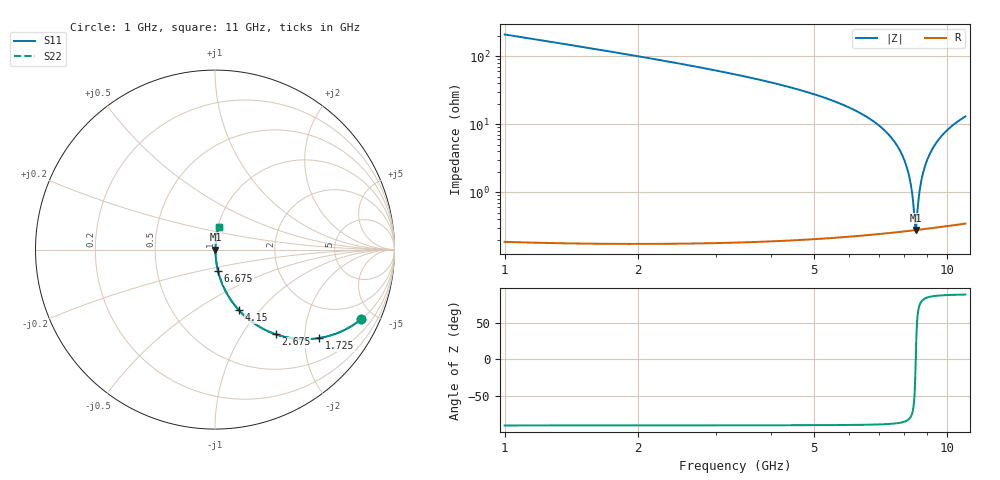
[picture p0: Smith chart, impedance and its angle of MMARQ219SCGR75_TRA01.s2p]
! MMARQ219SCGR75_TRA01  S-PARAMETER MODEL  ( General Type )
! Model Generated by TAIYO YUDEN Corporation (http://www.ty-top.com)
! Version 1.0
! TAIYO YUDEN Control No. 180601
! Copyright(c) 2018 TAIYO YUDEN CO.,LTD. All Rights Reserved.
! Product Description (link to TY-COMPAS)
! https://ds.yuden.co.jp/TYCOMPAS/or/detail?pn=MMARQ219SCGR75BTRA01&u=M
! Products Name : Multilayer Ceramic Capacitors
! Characteristics :
!  Capacitance : 0.75 pF , Rated Voltage : 250V , TCC : CG / C0G
!  Case Size : 2.0 x 1.25 / 0.079 x 0.049 [mm/inch] , Thickness : 0.85 / 0.033 [mm/inch]
!  (Conditions: Temperature = 25 degC , DC Bias Current/Voltage = 0A / 0V)
! External Node Assignments :
!  1  o---| |---o  2
! GND o---------o GND
! Frequency Range : 1000MHz  -  11000MHz  [ 401 STEP ]
# MHz S RI R 50
! Freq[MHz].  S11 Real  S11 Imag  S21 Real  S21 Imag  S12 Real  S12 Imag  S22 Real  S22 Imag
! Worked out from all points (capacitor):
!   401 points, 1 GHz to 11 GHz, reference 50 ohm
!   read as one part in series: C = 750 fF near 1.05 GHz
!   lowest |Z| = 280 mohm at 8.5 GHz (marker M1)
!   series resonance near 8.495 GHz, so ESL is about 470 pH
!   S11 on the Smith chart (normalised r, x): 1 GHz: 1.00, -4.18; 1.725 GHz: 1.00, -2.36; 2.675 GHz: 1.00, -1.43; 4.15 GHz: 1.00, -0.78; 6.675 GHz: 1.00, -0.24; 11 GHz: 1.01, +0.26
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1000  0.8138 -0.3888  0.1862 0.3888  0.1862 0.3888  0.8138 -0.3888
1725  0.5816 -0.4926  0.4184 0.4926  0.4184 0.4926  0.5816 -0.4926
2675  0.3383 -0.4719  0.6617 0.4719  0.6617 0.4719  0.3383 -0.4719
4150  0.1327 -0.3368  0.8673 0.3368  0.8673 0.3368  0.1327 -0.3368
4350  0.1159 -0.3174  0.8841 0.3174  0.8841 0.3174  0.1159 -0.3174
6000  0.0324 -0.171  0.9676 0.171  0.9676 0.171  0.0324 -0.171
6675  0.0168 -0.1192  0.9832 0.1192  0.9832 0.1192  0.0168 -0.1192
7250  0.0087 -0.0785  0.9913 0.0785  0.9913 0.0785  0.0087 -0.0785
7675  0.00512 -0.0503  0.9949 0.0503  0.9949 0.0503  0.00512 -0.0503
7975  0.00363 -0.0313  0.9964 0.0313  0.9964 0.0313  0.00363 -0.0313
8175  0.00306 -0.019  0.9969 0.019  0.9969 0.019  0.00306 -0.019
8300  0.00286 -0.0115  0.9971 0.0115  0.9971 0.0115  0.00286 -0.0115
8375  0.00279 -0.00703  0.9972 0.00703  0.9972 0.00703  0.00279 -0.00703
8450  0.00277 -0.00261  0.9972 0.00261  0.9972 0.00261  0.00277 -0.00261
8500  0.00278 0.000321  0.9972 -0.000321  0.9972 -0.000321  0.00278 0.000321
8550  0.0028 0.00323  0.9972 -0.00323  0.9972 -0.00323  0.0028 0.00323
8675  0.00293 0.0104  0.9971 -0.0104  0.9971 -0.0104  0.00293 0.0104
8800  0.00316 0.0175  0.9968 -0.0175  0.9968 -0.0175  0.00316 0.0175
9025  0.00382 0.03  0.9962 -0.03  0.9962 -0.03  0.00382 0.03
9350  0.00527 0.0475  0.9947 -0.0475  0.9947 -0.0475  0.00527 0.0475
10025  0.00995 0.0819  0.99 -0.0819  0.99 -0.0819  0.00995 0.0819
11000  0.02 0.1272  0.98 -0.1272  0.98 -0.1272  0.02 0.1272
